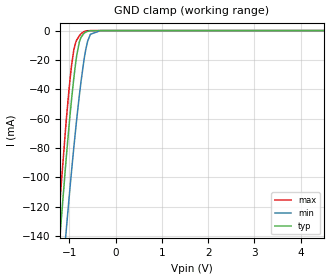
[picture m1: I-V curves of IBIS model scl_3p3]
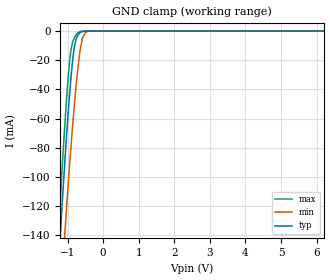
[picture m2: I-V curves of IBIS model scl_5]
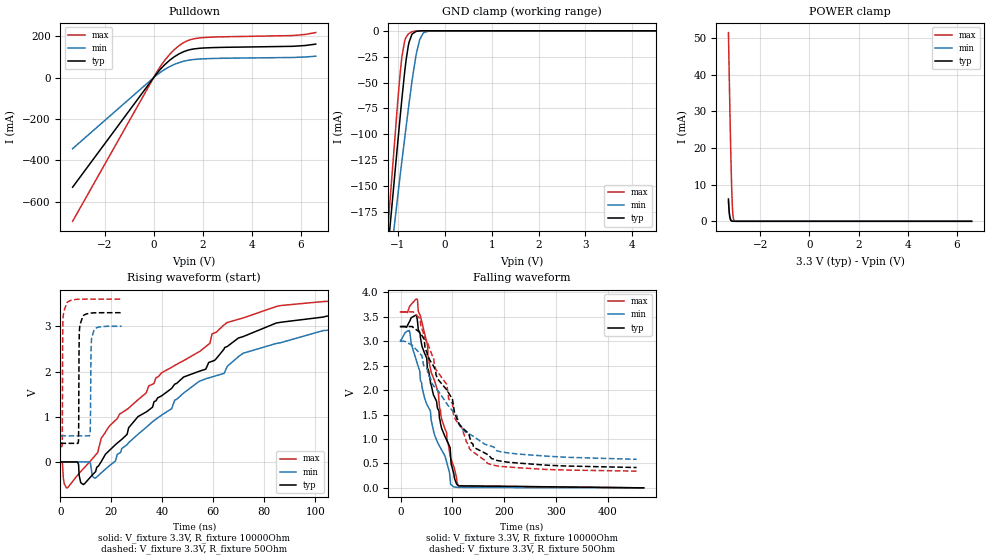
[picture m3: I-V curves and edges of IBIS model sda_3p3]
|Texas Instruments Incorporated
| Low Power, High Accuracy Humidity Sensor with Integrated Digital Temperature
| Sensor
| Marketing part#   Digital Voltage Range   Package-type   #pins
| HDC1080DMB   2.7V-5.5V   WSON   6
[IBIS Ver]   4.1
[File name]   hdc1080.ibs
[File Rev]   1.0
[Date]   12/11/2015
[Source]
| Texas Instruments Incorporated.
| Analog-eLab Design Center, HPA
| 12500 TI Blvd
| Dallas, TX -75243
[Notes]   Revision History:
| Rev 1.0: 12/11/2015
| - Replacement for HDC1050 model. Same buffer models
| - Initial version of the model
| - Model generated from simulations in SPECTRE
| - Model matched to SPICE simulation
| - C_comp although listed in numerical order of value are
|   obtained from varying PVT conditions. For PVT conditions for
|   each specific value refer the buffer description under
|   respective [Model]. IBIS model user is responsible for using
|   appropriate C_comp to simulate for Signal Integrity.
[Disclaimer]
| This model is designed as an aid for customers of Texas Instruments.
| TI and its licensors and suppliers make no warranties, either expressed
| or implied, with respect to this  model, including the warranties of
| merchantability or fitness for a particular purpose. The model is
| provided solely on an "as is" basis. The entire risk as to its quality
| and performance is with the customer.
[Copyright]
(C) Copyright 2015 Texas Instruments Incorporated.All rights reserved.
|   HDC1080DMB
[Component]   HDC1080DMB
[Manufacturer]   TI
[Package]   |6 PWSON  -  DMB package
|   typ   min   max
R_pkg   0.00500   0.00500   0.00500
L_pkg   0.20000nH   0.20000nH   0.20000nH
C_pkg   0.60000pF   0.60000pF   0.60000pF
[Pin]  signal_name   model_name   R_pin   L_pin   C_pin
1   SDA   SDA   0.00500   0.20000nH  0.60000pF
2   GND   GND   0.00500   0.20000nH  0.60000pF
3   NC   NC   0.00500   0.20000nH  0.60000pF
4   NC   NC   0.00500   0.20000nH  0.60000pF
5   VDD   POWER   0.00500   0.20000nH  0.60000pF
6   SCL   SCL   0.00500   0.20000nH  0.60000pF
|   Model Selectors
[Model Selector] SCL
scl_3p3   3.3V  digital Input
scl_5   5.0V  digital Input
[Model Selector] SDA
sda_3p3   3.3V digital I/O_open_drain
sda_5   5.0V digital I/O_open_drain
| Models and submodels in the file (4): scl_3p3 (Input), scl_5 (Input), sda_3p3 (I/O_open_drain), sda_5 (I/O_open_drain)
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|   scl_3p3 Model
[Model]   scl_3p3
Model_type   Input
Vinl = 0.99
Vinh = 2.31
|   typ   min   max
|   (nom PVT)   (fast PVT)   (slow PVT)
C_comp   4.581e-13   4.355e-13   5.484e-13
[Model spec]
|subparameter
Vinl   0.99   0.90   1.08
Vinh   2.31   2.10   2.52
| Where nom  PVT is Nominal Process, 3.3V, 27C
|   Fast PVT is Strong Process,  3.6V, -40C
|   Slow PVT is Weak Process,   3V, 150C
[Voltage Range]   3.3   3   3.6
|Junction Temperature
[Temperature Range]   27   150   -40
[Power Clamp Reference]   3.3   3   3.6
[GND Clamp Reference]   0   0   0
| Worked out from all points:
|   GND clamp passes 1 mA (typ) near -0.64 V on its own axis
[GND Clamp]
|   Voltage   I(typ)   I(min)   I(max)
-3.3V     -1.109A    -1.088A    -1.129A
-1.302V   -181.8mA   -225.7mA   -160.1mA
-1.188V   -134mA     -181mA     -109.9mA
-1.066V   -85.94mA   -135.2mA   -60.51mA
-980.1mV  -55.59mA   -104.8mA   -31.43mA
-906mV    -32.85mA   -80.22mA   -13.47mA
-785.4mV  -7.811mA   -44.37mA   -3.524mA
-686.4mV  -1.93mA    -20.42mA   -731.1uA
-606mV    -488.1uA   -7.307mA   -98.06uA
-546mV    -131.1uA   -2.528mA   -16.03uA
-330mV    -332.2nA   -27.49uA   0A
6.6V      0A         0A         0A
[POWER Clamp]
|   Voltage   I(typ)   I(min)   I(max)
-3.3V     0A         0A         0A
0V        0A         0A         0A
6.6V      0A         0A         0A
|   scl_5 Model
[Model]   scl_5
Model_type   Input
Vinl = 1.5
Vinh = 3.5
|   typ   min   max
|   (nom PVT)   (fast PVT)   (slow PVT)
C_comp   4.581e-13   4.355e-13   5.484e-13
[Model spec]
|subparameter
Vinl   1.5   1.35   1.65
Vinh   3.5   3.15   3.85
| Where nom  PVT is Nominal Process, 5V, 27C
|   Fast PVT is Strong Process,  5.5V, -40C
|   Slow PVT is Weak Process,   4.5V, 150C
[Voltage Range]   5   4.5   5.5
|Junction Temperature
[Temperature Range]   27   150   -40
[Power Clamp Reference]   5   4.5   5.5
[GND Clamp Reference]   0   0   0
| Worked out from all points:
|   GND clamp passes 1 mA (typ) near -0.64 V on its own axis
[GND Clamp]
|   Voltage   I(typ)   I(min)   I(max)
-5V       -1.919A    -1.85A     -1.968A
-1.288V   -174.9mA   -219.3mA   -152.8mA
-1.224V   -148.4mA   -194.6mA   -124.8mA
-1.12V    -106mA     -154.7mA   -80.8mA
-1.04V    -75.79mA   -125.4mA   -50.41mA
-940mV    -42.29mA   -90.81mA   -20.1mA
-860mV    -20.61mA   -65.41mA   -7.611mA
-800mV    -9.43mA    -47.96mA   -4.074mA
-660.5mV  -1.264mA   -15.15mA   -391.6uA
-585.5mV  -307.9uA   -5.078mA   -51.23uA
-365mV    -932.9nA   -57.1uA    -19.24nA
10V       0A         0A         0A
[POWER Clamp]
|   Voltage   I(typ)   I(min)   I(max)
-5V       0A         0A         0A
0V        0A         0A         0A
10V       0A         0A         0A
|   sda_3p3 Model
[Model]   sda_3p3
Model_type   I/O_open_drain
Polarity   Non-Inverting
Vinl = 0.99
Vinh = 2.31
Vmeas = 1.65
Vref = 3.3
Cref = 2pF
Rref = 10000
|   typ   min   max
|   (nom PVT)   (fast PVT)   (slow PVT)
C_comp   3.656e-12   3.601e-12   3.702e-12
[Model spec]
|subparameter
Vinl   0.99   0.90   1.08
Vinh   2.31   2.10   2.52
| Where nom  PVT is Nominal Process, 3.3V, 27C
|   Fast PVT is Strong Process,  3.6V, -40C
|   Slow PVT is Weak Process,   3V, 150C
[Voltage Range]   3.3   3   3.6
|Junction Temperature
[Temperature Range]   27   150   -40
[Pullup Reference]   3.3   3   3.6
[Pulldown Reference]   0   0   0
[Power Clamp Reference]   3.3   3   3.6
[GND Clamp Reference]   0   0   0
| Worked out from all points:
|   slope of the pulldown table from 0 to 0.495 V, typ, clamps not added: 7.34 ohm
|   GND clamp passes 1 mA (typ) near -0.62 V on its own axis
|   POWER clamp passes 1 mA (typ) near -3.24 V on its own axis
|   falling waveform, V_fixture 3.3V, R_fixture 10000Ohm: 20-80 % time 45.9ns typ, 50.3ns min, 42.4ns max; typ from 3.3 V to 0.002 V
|   rising waveform, V_fixture 3.3V, R_fixture 10000Ohm: 20-80 % time 41ns typ, 41.8ns min, 43ns max; typ from 0.002 V to 3.29 V
|   falling waveform, V_fixture 3.3V, R_fixture 50Ohm: 20-80 % time 83ns typ, 94.1ns min, 72.7ns max; typ from 3.3 V to 0.418 V
|   rising waveform, V_fixture 3.3V, R_fixture 50Ohm: 20-80 % time 180ps typ, 254ps min, 157ps max; typ from 0.413 V to 3.3 V
[Pulldown]
|   Voltage   I(typ)   I(min)   I(max)
-3.3V     -529mA     -342.9mA   -693.7mA
134.4mV   21.17mA    13.45mA    28.23mA
432mV     60.41mA    38.38mA    80.64mA
652.8mV   84.1mA     53.37mA    112.6mA
1.031V    114.6mA    72.51mA    154.3mA
1.442V    134.1mA    84.69mA    181.3mA
1.905V    142.3mA    90.36mA    192.5mA
5.655V    151.4mA    97.44mA    203.4mA
6.6V      162mA      103.5mA    217.8mA
[GND Clamp]
|   Voltage   I(typ)   I(min)   I(max)
-3.3V     -1.065A    -981.4mA   -1.128A
-1.381V   -296.3mA   -310mA     -290.7mA
-1.007V   -111.2mA   -162.5mA   -72.05mA
-913.2mV  -66.42mA   -126.4mA   -25.74mA
-852mV    -39.51mA   -103.8mA   -9.648mA
-776.4mV  -14.75mA   -76.39mA   -3.214mA
-699mV    -3.563mA   -49.56mA   -929.7uA
-609mV    -571.8uA   -23.07mA   -104uA
-534mV    -101.2uA   -8.759mA   -10.44uA
-453mV    -12.35uA   -1.907mA   -596.2nA
-330mV    -322nA     -97.28uA   0A
6.6V      0A         0A         0A
[POWER Clamp]
|   Voltage   I(typ)   I(min)   I(max)
-3.3V     6.079mA    5.422mA    51.48mA
-3.285V   4.075mA    3.945mA    45.96mA
-3.26V    1.908mA    2.239mA    37.15mA
-3.237V   849uA      1.253mA    29.12mA
-3.216V   393.1uA    727.4uA    22.33mA
-3.185V   120.4uA    316.3uA    13.31mA
-3.163V   52.62uA    175.5uA    8.179mA
-3.142V   22.84uA    96.55uA    4.338mA
-3.12V    9.942uA    52.54uA    1.948mA
-3.098V   4.309uA    28.13uA    761.6uA
-3.052V   706.8nA    6.22uA     80.17uA
6.6V      0A         0A         0A
[Ramp]
R_load = 10000
|   typ   min   max
dV/dt_r   1.97842/4.12082e-08   1.81097/4.18779e-08   2.15873/4.2809e-08
dV/dt_f   1.97871/4.58818e-08   1.81135/5.0703e-08   2.15892/4.26244e-08
[Falling Waveform]
V_fixture = 3.3V
V_fixture_min = 3V
V_fixture_max = 3.6V
R_fixture = 10000Ohm
|   Time   V(typ)   V(min)   V(max)
0s        3.3V       3V         3.6V
17.14ns   3.401V     3.22V      3.703V
32.81ns   3.394V     2.527V     3.843V
52.17ns   2.446V     1.681V     2.909V
58.81ns   2.116V     1.419V     2.37V
65.24ns   1.864V     1.095V     2.202V
85.73ns   1.05V      652.1mV    1.205V
96.73ns   622.9mV    66.66mV    610.4mV
112.4ns   42.62mV    9.34mV     42.82mV
468.7ns   2.071mV    2.983mV    1.698mV
[Rising Waveform]
V_fixture = 3.3V
V_fixture_min = 3V
V_fixture_max = 3.6V
R_fixture = 10000Ohm
|   Time   V(typ)   V(min)   V(max)
0s        2.049mV    2.948mV    1.682mV
2.327ns   2.049mV    2.948mV    -570.8mV
6.631ns   2.209mV    2.948mV    -295.6mV
9.006ns   -498.3mV   2.948mV    -147.5mV
13.9ns    -190.1mV   -346.6mV   163.6mV
23.19ns   459.8mV    196.8mV    1.059V
38.22ns   1.421V     976.7mV    1.881V
65.31ns   2.55V      2.091V     3.08V
103.2ns   3.204V     2.906V     3.547V
158.3ns   3.294V     3.012V     3.596V
[Falling Waveform]
V_fixture = 3.3V
V_fixture_min = 3V
V_fixture_max = 3.6V
R_fixture = 50Ohm
|   Time   V(typ)   V(min)   V(max)
0s        3.3V       3V         3.6V
37.76ns   3.177V     2.743V     3.458V
67.7ns    2.391V     2.037V     2.432V
89.11ns   2.005V     1.726V     2.119V
100ns     1.814V     1.579V     1.726V
103.9ns   1.562V     1.533V     1.442V
132.5ns   1.069V     1.101V     808.2mV
142.5ns   823.2mV    1.04V      716.5mV
168.4ns   678.9mV    874.3mV    497.8mV
455ns     417.7mV    584.9mV    344mV
[Rising Waveform]
V_fixture = 3.3V
V_fixture_min = 3V
V_fixture_max = 3.6V
R_fixture = 50Ohm
|   Time   V(typ)   V(min)   V(max)
0s        412.8mV    578.3mV    341mV
676ps     412.8mV    578.3mV    374.5mV
983ps     412.8mV    578.3mV    3.139V
2.222ns   412.8mV    578.3mV    3.492V
7.082ns   461.8mV    578.3mV    3.597V
7.425ns   2.885V     578.3mV    3.598V
8.577ns   3.197V     578.3mV    3.599V
11.65ns   3.289V     640.6mV    3.6V
13.15ns   3.297V     2.91V      3.6V
24.04ns   3.3V       3V         3.6V
